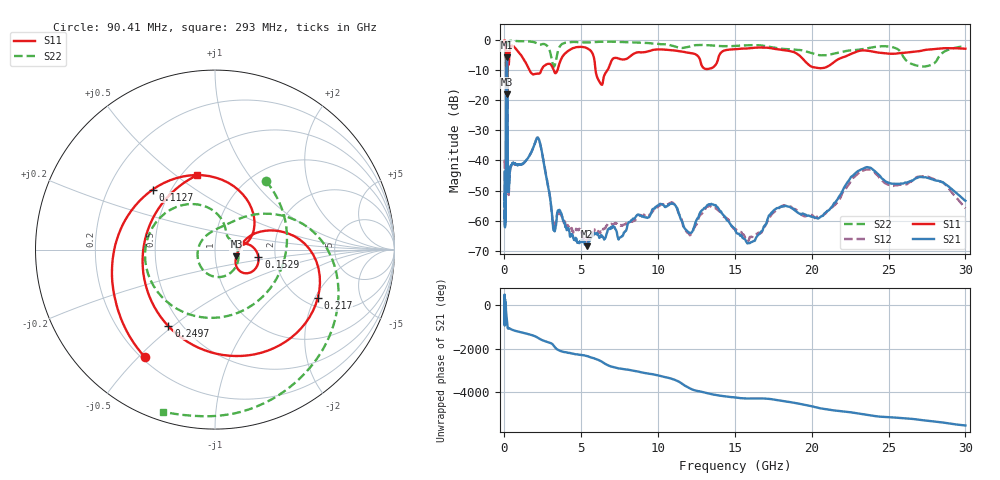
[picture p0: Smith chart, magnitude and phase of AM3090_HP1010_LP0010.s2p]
! Date/Time: Thu, Feb 28, 2019 2:04 PM
! Network Analyzer: Agilent Technologies E8364B Rev: A.07.50.67
! Sweep from 0.010 to 30.000 GHz, 1601 Points, Sweep Type: LOG
! Power Supply: 5.022 V, 0.002 A
# Hz S DB R 50
!freq MagS11 AngS11 MagS21 AngS21 MagS12 AngS12 MagS22 AngS22
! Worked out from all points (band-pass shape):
!   1601 points, 10 MHz to 30 GHz, reference 50 ohm
!   highest |S21| = -5.71 dB at 152.1 MHz (marker M1); lowest = -68.4 dB at 5.365 GHz (marker M2)
!   |S21| within 3 dB of the highest: 126.2 MHz to 187.4 MHz (61.12 MHz wide, 39 % of centre)
!   lowest |S11| = -18.1 dB at 184.9 MHz (marker M3), VSWR 1.29, Z = 63.3 - j4.73 ohm
!   |S11| at or under -10 dB: 1.618 GHz to 2.401 GHz (782.6 MHz wide, 38.9 % of centre); 3.2 GHz to 3.453 GHz (252.6 MHz wide, 7.59 % of centre); 5.927 GHz to 6.709 GHz (782.3 MHz wide, 12.4 % of centre)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
!   |S22| runs from -21.0 to -0.2 dB; largest |S21 - S12| = 0.015
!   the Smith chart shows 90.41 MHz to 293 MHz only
!   S11 on the Smith chart (normalised r, x): 90.41 MHz: 0.21, -0.52; 112.7 MHz: 0.40, +0.35; 152.9 MHz: 1.63, -0.14; 217 MHz: 2.36, -2.11; 249.7 MHz: 0.42, -0.48; 293 MHz: 0.59, +0.60
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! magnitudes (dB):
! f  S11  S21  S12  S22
! 10 MHz  -0.2  -43.8  -39.8  -0.6
! 38.04 MHz  -0.5  -57.0  -60.2  -1.3
! 49.59 MHz  -0.7  -50.5  -48.6  -1.4
! 90.41 MHz  -2.9  -52.1  -50.9  -6.4
! 112.7 MHz  -6.3  -21.5  -21.5  -8.0
! 144.7 MHz  -13.9  -5.8  -5.8  -18.6
! 152.1 MHz  -12.3  -5.7  -5.7  -16.7
! 152.9 MHz  -12.2  -5.7  -5.7  -16.6
! 184.9 MHz  -18.1  -8.1  -8.0  -19.6
! 217 MHz  -4.0  -43.9  -44.0  -2.7
! 249.7 MHz  -6.0  -50.0  -49.8  -0.9
! 293 MHz  -7.4  -49.0  -49.9  -0.5
! 550.5 MHz  -2.1  -40.9  -41.0  -0.3
! 2.084 GHz  -11.2  -32.9  -32.9  -1.0
! 3.22 GHz  -10.3  -63.2  -62.3  -8.9
! 5.365 GHz  -2.7  -68.4  -66.2  -0.8
! 6.234 GHz  -14.3  -65.5  -64.1  -0.6
! 7.926 GHz  -6.3  -63.2  -60.8  -0.7
! 13.47 GHz  -9.4  -54.4  -55.4  -1.8
! 16.05 GHz  -2.7  -67.1  -65.3  -1.7
! 23.48 GHz  -3.5  -42.4  -43.0  -2.9
! 30 GHz  -2.9  -53.4  -55.9  -2.2
